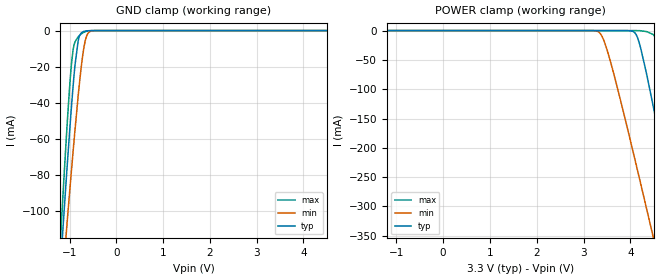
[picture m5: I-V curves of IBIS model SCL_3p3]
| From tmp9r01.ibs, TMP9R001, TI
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|   Model
[Model]   SCL_3p3
Model_type   Input
Vinl = 0.99
Vinh = 2.31
|   typ   min   max
C_comp   0.826pF   0.806pF   0.832pF
[Voltage Range]   3.3   2.7   3.6
[Temperature Range]   25   125   -40
[Power Clamp Reference]   3.3   2.7   3.6
[GND Clamp Reference]   0   0   0
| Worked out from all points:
|   GND clamp passes 1 mA (typ) near -0.73 V on its own axis
[GND Clamp]
|   Voltage   I(typ)   I(min)   I(max)
-3.3V     -1.018A    -874mA     -1.169A
-1.181V   -126.1mA   -148.4mA   -110.3mA
-1.122V   -102.7mA   -129.1mA   -83.12mA
-1.063V   -79.94mA   -110.1mA   -57.08mA
-1.003V   -57.98mA   -91.4mA    -33.33mA
-953.7mV  -40.71mA   -76.16mA   -17.35mA
-904.2mV  -25.07mA   -61.34mA   -8.078mA
-815.1mV  -5.689mA   -36.3mA    -3.443mA
-706.2mV  -597.3uA   -11.73mA   -1.117mA
-617.1mV  -113.1uA   -2.044mA   -250.4uA
-468.6mV  -4.071uA   -38.51uA   -6.681uA
6.6V      0A         0A         0A
[POWER Clamp]
|   Voltage   I(typ)   I(min)   I(max)
-3.3V     0A         0A         0A
3.313V    -14.36nA   -1.86mA    -13.57nA
3.551V    -23.77nA   -46.01mA   -14.26nA
4.095V    -3.66mA    -219.1mA   -14.01uA
4.363V    -79.94mA   -309.2mA   -2.15mA
4.491V    -130mA     -352.9mA   -6.841mA
4.6V      -173.8mA   -390.1mA   -32.23mA
4.848V    -275.5mA   -475mA     -141.5mA
5.075V    -370.5mA   -553.5mA   -251.8mA
5.204V    -424.6mA   -597.9mA   -315.3mA
5.432V    -520.7mA   -676.7mA   -428.5mA
6.6V      -1.018A    -1.083A    -1.017A
